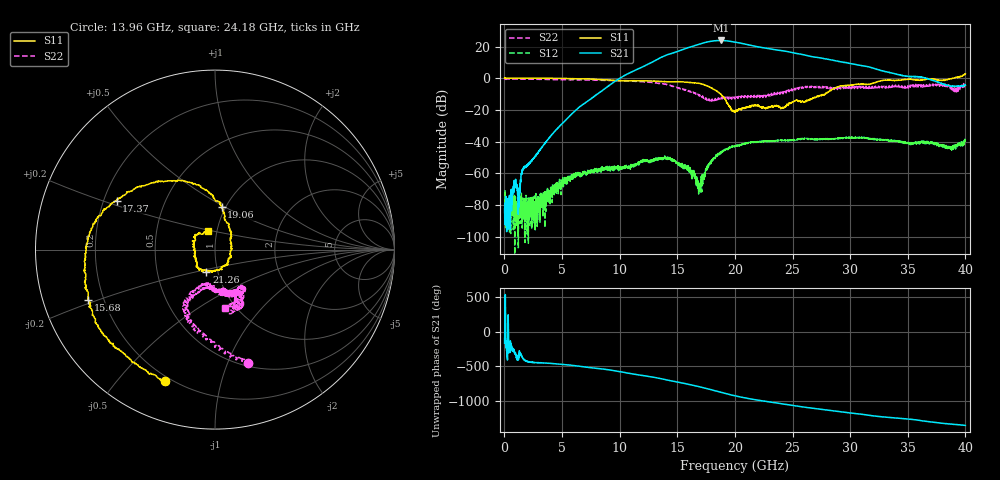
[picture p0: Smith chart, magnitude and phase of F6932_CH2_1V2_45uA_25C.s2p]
!Keysight Technologies,M9807A,MY58100526,A.15.20.05
!Date: Tuesday, August 01, 2023 09:07:37
!Correction: S11(Cdelta 2-Port  )
!S21(Cdelta 2-Port  )
!S12(Cdelta 2-Port  )
!S22(Cdelta 2-Port  )
!S2P File: Measurements: S11, S21, S12, S22:
# Hz S  dB  R 50
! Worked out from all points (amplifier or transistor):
!   4000 points, 10 MHz to 40 GHz, reference 50 ohm
!   highest |S21| = 23.9 dB at 18.82 GHz (marker M1)
!   |S21| within 3 dB of that: 16.62 GHz to 21.33 GHz (4.706 GHz wide, 24.8 % of centre)
!   unconditionally stable (mu >= 1): 79.66 MHz to 140.4 MHz; 339.7 MHz to 430.3 MHz; 4.02 GHz to 38.88 GHz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
!   at 6.67 GHz: K = 65.73, MAG = 0.3 dB, |S12| = -60.2 dB
!   at 20.01 GHz: K = 4.70, MAG = 23.1 dB, |S12| = -42.8 dB
!   at 40 GHz: K = -40.52, MSG = 17.7 dB, |S12| = -39.7 dB
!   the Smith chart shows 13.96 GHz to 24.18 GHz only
!   S11 on the Smith chart (normalised r, x): 13.96 GHz: 0.18, -0.67; 15.68 GHz: 0.14, -0.19; 17.37 GHz: 0.25, +0.22; 19.06 GHz: 0.96, +0.48; 21.26 GHz: 0.88, -0.22; 24.18 GHz: 0.90, +0.19
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1e7  0.07 178.3  -82.37 -164.5  -80.16 -93.8  -0.77 178.1
6.68e9  -0.37 68.1  -17.22 -144.8  -59.72 144.9  -1.01 62.3
1.09e10  -1.57 -36.8  3.56 115.5  -55.95 91.6  -1.62 -14.2
1.334e10  -1.90 -90.0  12.24 48.7  -50.73 55.9  -3.17 -59.0
1.396e10  -2.11 -110.9  14.42 26.5  -50.62 34.8  -3.68 -73.9
1.568e10  -2.37 -158.5  18.69 -31.5  -54.68 -3.2  -7.40 -110.5
1.657e10  -2.95 176.5  20.80 -63.7  -61.93 -51.3  -9.67 -117.0
1.737e10  -4.26 153.5  22.52 -95.0  -59.60 160.0  -12.56 -109.3
1.806e10  -6.57 126.0  23.53 -125.6  -51.85 120.8  -13.88 -94.4
1.882e10  -10.38 92.2  23.91 -159.8  -46.63 97.6  -12.16 -84.8
1.906e10  -12.43 81.2  23.80 -170.4  -45.22 90.1  -12.65 -82.6
1.947e10  -17.37 50.3  23.48 172.0  -44.19 73.7  -12.62 -82.3
2.001e10  -21.33 -16.5  22.85 151.1  -42.80 57.0  -12.63 -81.7
2.061e10  -18.80 -72.1  22.00 129.9  -41.69 41.9  -11.32 -69.8
2.126e10  -17.63 -111.6  20.99 109.3  -40.76 24.7  -10.99 -66.7
2.267e10  -19.20 -175.9  19.02 70.8  -39.45 -5.1  -11.72 -56.1
2.418e10  -18.89 111.0  17.36 32.4  -38.94 -33.3  -9.64 -79.8
2.667e10  -12.96 9.6  13.69 -27.1  -38.38 -78.6  -5.06 -92.8
2.829e10  -7.78 -42.9  11.70 -62.3  -38.53 -101.8  -5.74 -98.6
3.025e10  -4.24 -73.0  8.98 -102.2  -37.50 -132.5  -6.45 -123.7
3.334e10  -1.19 -128.8  3.77 -162.2  -39.13 171.5  -5.73 -158.4
4e10  2.84 114.3  -4.39 81.8  -39.73 48.6  -3.46 116.5
